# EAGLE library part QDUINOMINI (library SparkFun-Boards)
Qduino Mini Board Outline and Pins Board outline for SparkFun Qduino Mini
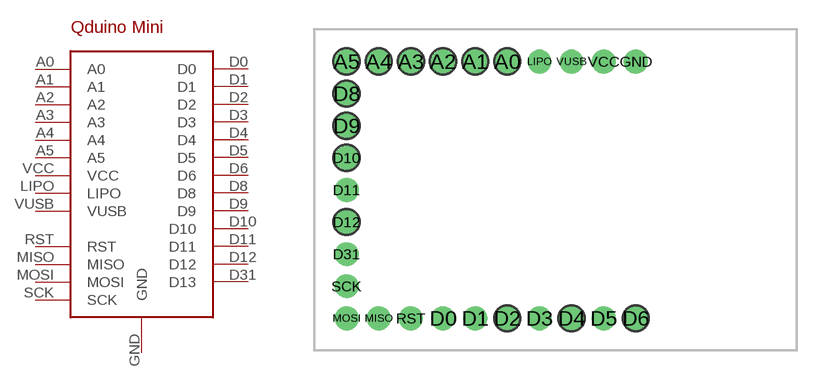
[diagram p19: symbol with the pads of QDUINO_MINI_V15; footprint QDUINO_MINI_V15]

Designator prefix BOARD

## QDUINOMINI  [QDUINO_MINI_V15]
A0  A0
A1  A1
A2  A2
A3  A3
A4  A4
A5  A5
D0  D0
D1  D1
D2  D2
D3  D3
D4  D4
D5  D5
D6  D6
D8  D8
D9  D9
D10  D10
D11  D11
D12  D12
D31  D13
GND  GND
LIPO  LIPO
MISO  MISO
MOSI  MOSI
RST  RST
SCK  SCK
VCC  VCC
VUSB  VUSB

## Footprint QDUINO_MINI_V15 (pad centres in mm)
Qduino Mini Board Outline and Pins Board outline for SparkFun Qduino Mini Devices using: QDUINOMINI
drill 1.016 pad 1.88: A0 -3.81,10.16; A1 -6.35,10.16; A2 -8.89,10.16; A3 -11.43,10.16; A4 -13.97,10.16; A5 -16.51,10.16; D0 -8.89,-10.16; D1 -6.35,-10.16; D2 -3.81,-10.16; D3 -1.27,-10.16; D4 1.27,-10.16; D5 3.81,-10.16; D6 6.35,-10.16; D8 -16.51,7.62; D9 -16.51,5.08; D10 -16.51,2.54; D11 -16.51,0; D12 -16.51,-2.54; D31 -16.51,-5.08; GND 6.35,10.16; LIPO -1.27,10.16; MISO -13.97,-10.16; MOSI -16.51,-10.16; RST -11.43,-10.16; SCK -16.51,-7.62; VCC 3.81,10.16; VUSB 1.27,10.16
